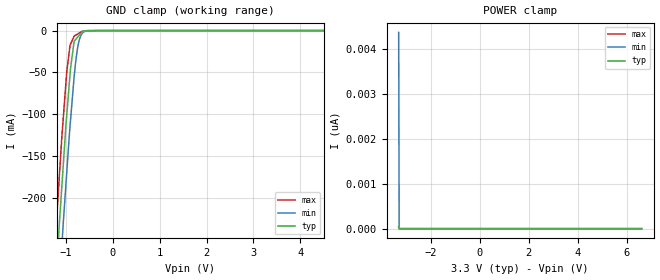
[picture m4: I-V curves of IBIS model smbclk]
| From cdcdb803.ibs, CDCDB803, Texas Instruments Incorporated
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[Model]   smbclk
Model_type   Input
Vinl = 0.66
Vinh = 2.64
|   typ   min   max
C_comp   0.6p   0.5p   0.7p
|  Where Nom  PVT is Nominal Process, 3.3V,   32C
|   Fast PVT is Strong Process,  3.465V, -35C
|   Slow PVT is Weak Process,   3.135V,  110C
[Model spec]
|subparameter
Vinl   0.66   0.627   0.693
Vinh   2.64   2.508   2.772
[Voltage Range]   3.3   3.135   3.465
|Junction Temperature
[Temperature Range]   27   125   -40
[Power Clamp Reference]   3.3   3.135   3.465
[GND Clamp Reference]   0   0   0
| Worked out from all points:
|   GND clamp passes 1 mA (typ) near -0.65 V on its own axis
[GND Clamp]
|   Voltage   I(typ)   I(min)   I(max)
-3.3V     -2.319A    -2.382A    -2.268A
-1.247V   -327.9mA   -403.1mA   -267.9mA
-1.146V   -236.1mA   -311.5mA   -179.3mA
-1.087V   -186.9mA   -258.2mA   -127.8mA
-1.055V   -159.9mA   -229mA     -103.9mA
-982.4mV  -101.3mA   -170mA     -49.75mA
-901.4mV  -45.09mA   -107.1mA   -16.3mA
-824.2mV  -12.79mA   -54.9mA    -6.555mA
-768.1mV  -9.048mA   -27.28mA   -4.658mA
-712.6mV  -5.347mA   -10.81mA   -2.799mA
-642mV    -630.8uA   -2.787mA   -774.6uA
6.6V      0A         0A         0A
[POWER Clamp]
|   Voltage   I(typ)   I(min)   I(max)
-3.3V     45.09pA    4.378nA    27.16pA
-3.28V    0A         0A         0A
-3.27V    0A         0A         0A
6.6V      0A         0A         0A
